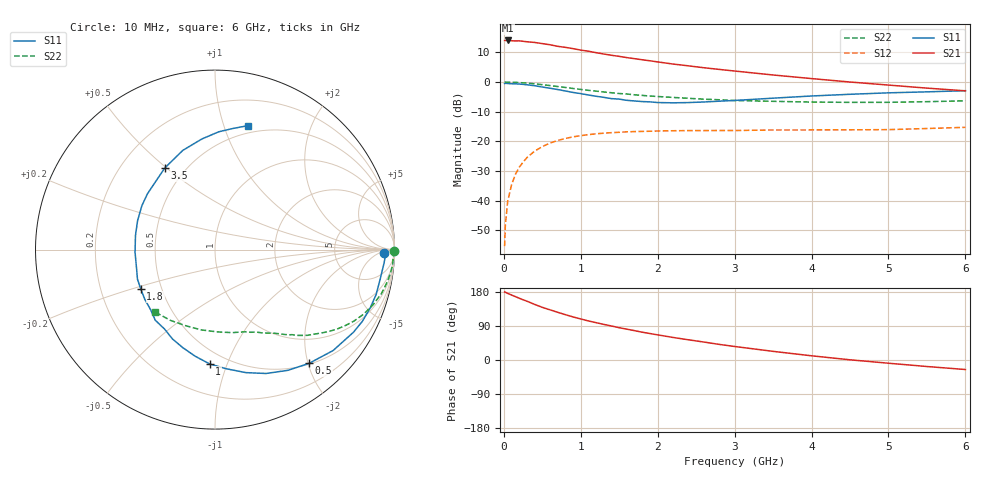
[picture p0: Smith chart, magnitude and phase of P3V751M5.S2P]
! SIEMENS Small Signal Semiconductors
! BFP181
! Si NPN RF Bipolar Junction Transistor in SOT143
! VCE = 0.75 V  IC = 1.5 mA
! Common Emitter S-Parameters:  March  1996
# GHz  S  MA  R  50
!  f  S11  S21  S12  S22
! GHz  MAG  ANG  MAG  ANG  MAG  ANG  MAG  ANG
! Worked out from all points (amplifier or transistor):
!   36 points, 10 MHz to 6 GHz, reference 50 ohm
!   highest |S21| = 14.0 dB at 50 MHz (marker M1)
!   |S21| within 3 dB of that: start of sweep to 949 MHz
!   unconditionally stable (mu >= 1): 2.466 GHz to end of sweep
!   at 250 MHz: K = 0.11, MSG = 20.4 dB, |S12| = -27.1 dB
!   at 1.4 GHz: K = 0.63, MSG = 13.1 dB, |S12| = -17.1 dB
!   at 6 GHz: K = 1.31, MAG = 2.8 dB, |S12| = -15.3 dB
!   S11 on the Smith chart (normalised r, x): 10 MHz: 30, -12; 500 MHz: 0.52, -2.02; 1 GHz: 0.40, -0.87; 1.8 GHz: 0.38, -0.21; 3.5 GHz: 0.39, +0.49; 6 GHz: 0.43, +1.21
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0.01  0.9441 -1.3  5.017 179.5  0.0017 86.5  0.9965 -0.4
0.02  0.9504 -2.1  5.017 178.9  0.0039 86.9  0.9947 -1.0
0.05  0.9437 -5.0  5.026 175.7  0.0097 89.2  0.9936 -2.6
0.1  0.9347 -10.3  4.973 171.5  0.0184 83.6  0.9929 -5.1
0.2  0.9236 -20.7  4.948 163.0  0.0364 77.1  0.9784 -10.1
0.4  0.8656 -40.5  4.652 146.7  0.0682 65.0  0.9324 -19.3
0.5  0.8225 -50.4  4.447 139.0  0.0814 59.0  0.9028 -23.5
0.6  0.7856 -58.9  4.252 132.4  0.0932 54.0  0.8709 -27.2
0.8  0.7067 -75.9  3.844 119.6  0.1115 45.2  0.8091 -33.3
0.9  0.6669 -84.6  3.659 113.7  0.1189 41.3  0.7779 -36.0
1  0.6376 -92.7  3.456 108.3  0.1242 37.9  0.7494 -38.4
1.1  0.6039 -100.6  3.307 103.0  0.1296 34.8  0.7236 -40.7
1.3  0.5512 -115.5  2.965 93.9  0.1369 29.0  0.6796 -44.7
1.5  0.5151 -130.3  2.71 85.2  0.1418 24.7  0.6397 -47.8
1.8  0.4679 -152.1  2.372 73.3  0.1468 19.7  0.5942 -52.2
2.2  0.4457 -178.1  2.01 59.5  0.1507 14.2  0.5495 -57.9
2.8  0.4751 149.1  1.632 41.2  0.152 8.7  0.5019 -66.6
3.5  0.534 121.6  1.314 22.8  0.1552 4.6  0.4724 -78.3
4  0.5811 108.0  1.143 11.1  0.1554 2.3  0.4587 -88.4
4.5  0.621 96.7  1 0.5  0.1561 0.5  0.4538 -99.5
5.5  0.6826 81.5  0.789 -17.2  0.1642 0.2  0.4659 -122.1
6  0.714 75.2  0.71 -25.1  0.172 -0.7  0.4816 -133.5
